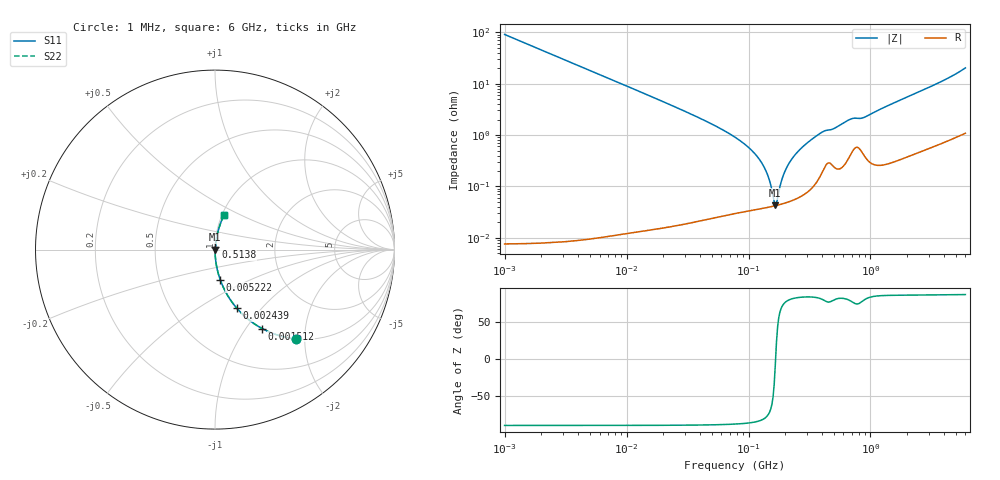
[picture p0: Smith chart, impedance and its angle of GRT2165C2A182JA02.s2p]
!Murata Part Number: GRT2165C2A182JA02
!These Parameters are Measured in Series Mode Connection
!Data Generated on Jun 19, 2026
!  o--ll--o
!Port1  Port2
!  o------o
!Operation Temp=25[degC], DC Bias Voltage=0[V]
!Freq. Start=1000[kHz] Stop=6[GHz] 401[Steps]
# Hz S RI R 50
!Freq.(Hz) S11(Real) S11(Imag) S21(Real) S21(Imag) S12(Real) S12(Imag) S22(Real) S22(Imag)
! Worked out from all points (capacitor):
!   401 points, 1 MHz to 6 GHz, reference 50 ohm
!   read as one part in series: C = 1.76 nF near 1.044 MHz
!   lowest |Z| = 42.6 mohm at 165.8 MHz (marker M1)
!   series resonance near 166.7 MHz, so ESL is about 520 pH
!   S11 on the Smith chart (normalised r, x): 1 MHz: 1.00, -1.80; 1.512 MHz: 1.00, -1.19; 2.439 MHz: 1.00, -0.74; 5.222 MHz: 1.00, -0.35; 513.8 MHz: 1.00, +0.03; 6 GHz: 1.02, +0.40
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1000000  0.4488 -0.4973  0.5512 0.4973  0.5512 0.4973  0.4488 -0.4973
1511688  0.2627 -0.4401  0.7373 0.4401  0.7373 0.4401  0.2627 -0.4401
2439274  0.1204 -0.3253  0.8796 0.3253  0.8796 0.3253  0.1204 -0.3253
4293785  0.0423 -0.2011  0.9577 0.2011  0.9577 0.2011  0.0423 -0.2011
5222143  0.029 -0.1676  0.971 0.1676  0.971 0.1676  0.029 -0.1676
1.843659e7  0.00248 -0.0481  0.9975 0.0481  0.9975 0.0481  0.00248 -0.0481
7.745967e7  0.000379 -0.00907  0.9996 0.00907  0.9996 0.00907  0.000379 -0.00907
1.050294e8  0.000366 -0.00514  0.9996 0.00514  0.9996 0.00514  0.000366 -0.00514
1.277378e8  0.000379 -0.0029  0.9996 0.0029  0.9996 0.0029  0.000379 -0.0029
1.424119e8  0.000393 -0.0017  0.9996 0.0017  0.9996 0.0017  0.000393 -0.0017
1.587717e8  0.000412 -0.000526  0.9996 0.000526  0.9996 0.000526  0.000412 -0.000526
1.658303e8  0.000422 -5.73e-05  0.9996 5.73e-05  0.9996 5.73e-05  0.000422 -5.73e-05
1.732027e8  0.000433 0.000412  0.9996 -0.000412  0.9996 -0.000412  0.000433 0.000412
1.930997e8  0.000468 0.00159  0.9995 -0.00159  0.9995 -0.00159  0.000468 0.00159
2.152823e8  0.000513 0.0028  0.9995 -0.0028  0.9995 -0.0028  0.000513 0.0028
2.561955e8  0.000624 0.00483  0.9994 -0.00483  0.9994 -0.00483  0.000624 0.00483
3.325952e8  0.00101 0.0083  0.999 -0.0083  0.999 -0.0083  0.00101 0.0083
5.138348e8  0.00246 0.0135  0.9975 -0.0135  0.9975 -0.0135  0.00246 0.0135
6.817316e8  0.00438 0.0197  0.9956 -0.0197  0.9956 -0.0197  0.00438 0.0197
8.8503e8  0.00445 0.0214  0.9955 -0.0214  0.9955 -0.0214  0.00445 0.0214
1.428092e9  0.00425 0.0381  0.9958 -0.0381  0.9958 -0.0381  0.00425 0.0381
6e9  0.0487 0.1901  0.9513 -0.1901  0.9513 -0.1901  0.0487 0.1901
